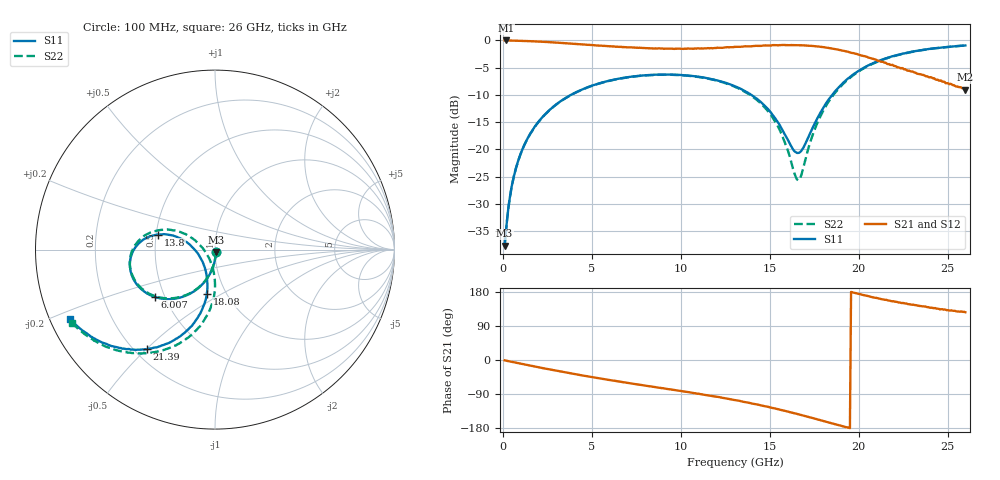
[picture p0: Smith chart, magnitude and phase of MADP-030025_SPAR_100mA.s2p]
!Mean
# HZ S DB R 50
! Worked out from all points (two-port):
!   400 points, 100 MHz to 26 GHz, reference 50 ohm
!   highest |S21| = -0.03 dB at 164.9 MHz (marker M1); lowest = -9.1 dB at 26 GHz (marker M2)
!   |S21| within 3 dB of the highest: start of sweep to 20.46 GHz
!   lowest |S11| = -37.6 dB at 100 MHz (marker M3), VSWR 1.03, Z = 50.4 - j1.26 ohm
!   |S11| at or under -10 dB: start of sweep to 3.828 GHz; 13.97 GHz to 18.51 GHz (4.543 GHz wide, 28 % of centre)
!   |S22| runs from -37.7 to -1.0 dB; largest |S21 - S12| = 0.0059
!   S11 on the Smith chart (normalised r, x): 100 MHz: 1.01, -0.03; 6.007 GHz: 0.44, -0.28; 13.8 GHz: 0.51, +0.10; 18.08 GHz: 0.81, -0.43; 21.39 GHz: 0.25, -0.50; 26 GHz: 0.06, -0.22
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1e8  -37.65 -72.7  -0.03 -0.8  -0.03 -0.8  -37.72 -74.0
1.6491e8  -35.42 -77.1  -0.03 -1.6  -0.04 -1.6  -35.36 -77.9
3.5965e8  -29.56 -84.8  -0.05 -3.5  -0.05 -3.5  -29.58 -84.8
6.193e8  -24.92 -90.0  -0.06 -6.1  -0.07 -6.1  -24.95 -90.5
1.3333e9  -18.32 -99.7  -0.12 -12.9  -0.13 -12.9  -18.37 -99.7
2.6316e9  -12.74 -113.0  -0.34 -24.9  -0.34 -24.9  -12.78 -113.3
4.4491e9  -9.02 -129.4  -0.75 -40.5  -0.74 -40.6  -9.05 -130.1
6.007e9  -7.39 -142.1  -1.09 -53.0  -1.10 -52.9  -7.41 -142.8
8.7982e9  -6.29 -162.3  -1.47 -73.2  -1.48 -73.3  -6.32 -163.7
1.1005e10  -6.67 -177.2  -1.47 -89.0  -1.48 -89.0  -6.72 -179.4
1.3082e10  -8.48 169.3  -1.20 -106.1  -1.22 -106.1  -8.57 165.2
1.3796e10  -9.65 165.3  -1.10 -112.5  -1.11 -112.6  -9.79 160.2
1.5419e10  -14.79 163.3  -0.89 -129.1  -0.89 -129.2  -15.51 152.5
1.6588e10  -20.64 -150.2  -0.91 -142.9  -0.91 -142.9  -25.66 -151.7
1.6782e10  -20.24 -134.7  -0.91 -145.3  -0.91 -145.3  -24.67 -123.3
1.7367e10  -16.37 -107.8  -1.02 -152.6  -1.02 -152.5  -17.81 -92.8
1.8081e10  -11.98 -100.5  -1.29 -161.8  -1.29 -161.8  -12.46 -90.5
1.9379e10  -7.05 -106.8  -2.07 -178.0  -2.06 -178.0  -7.21 -101.1
2.1391e10  -3.44 -124.5  -3.98 159.9  -3.97 160.0  -3.51 -121.0
2.1716e10  -3.11 -127.1  -4.36 156.7  -4.35 156.6  -3.16 -123.8
2.3858e10  -1.63 -142.7  -6.60 139.5  -6.61 139.5  -1.65 -140.4
2.6e10  -0.94 -154.6  -9.06 125.9  -8.93 125.9  -0.95 -153.0
